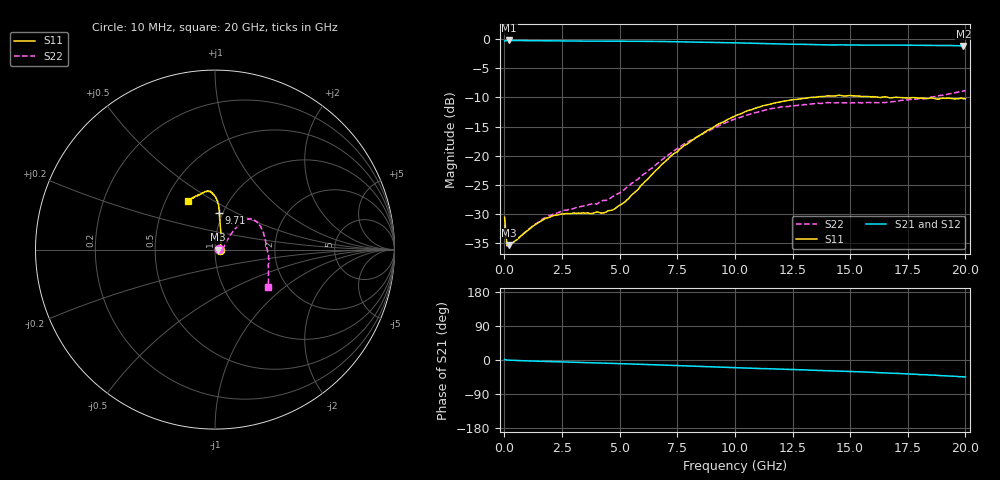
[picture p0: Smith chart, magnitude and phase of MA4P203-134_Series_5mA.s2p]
! AWR Design Environment (9226) Thu Aug 19 14:29:25 2021
! Document = '5mA'
! nPorts: 2, nXvals: 201
# GHz S DB R 50
!Freq DBS11 AngS11 DBS21 AngS21 DBS12 AngS12 DBS22 AngS22
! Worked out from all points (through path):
!   201 points, 10 MHz to 20 GHz, reference 50 ohm
!   highest |S21| = -0.20 dB at 210 MHz (marker M1); lowest = -1.1 dB at 19.91 GHz (marker M2)
!   group delay of S21, straight-line fit = 5.94 ps
!   lowest |S11| = -35.4 dB at 210 MHz (marker M3), VSWR 1.03, Z = 51.7 - j0.00352 ohm
!   |S11| at or under -10 dB: start of sweep to 13.27 GHz; 16.66 GHz to 16.89 GHz (226.5 MHz wide, 1.35 % of centre); 17.13 GHz to end of sweep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
!   |S22| runs from -35.6 to -8.8 dB; largest |S21 - S12| = 0.043
!   S11 on the Smith chart (normalised r, x): 10 MHz: 1.06, -0.00; 9.71 GHz: 0.96, +0.41; 20 GHz: 0.65, +0.39
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0.01  -30.60 -1.1  -0.28 1.4  -0.26 1.0  -31.91 11.3
0.11  -35.35 -2.9  -0.20 -0.2  -0.19 -0.2  -35.56 -3.5
0.21  -35.36 -0.1  -0.20 -0.5  -0.19 -0.5  -35.42 0.5
1.21  -32.21 -4.0  -0.25 -2.7  -0.23 -2.6  -32.14 -4.3
1.81  -30.76 -11.5  -0.28 -3.8  -0.26 -3.5  -30.57 -11.5
2.41  -30.09 -15.8  -0.29 -4.8  -0.28 -4.5  -29.67 -15.9
3.41  -29.83 -10.7  -0.31 -6.7  -0.29 -6.1  -28.66 -11.9
4.01  -29.67 -0.2  -0.31 -7.8  -0.30 -7.2  -28.35 -3.8
4.21  -29.90 6.7  -0.32 -8.1  -0.30 -7.5  -27.79 -1.1
4.81  -29.10 23.8  -0.33 -9.2  -0.31 -8.6  -26.84 8.9
5.31  -27.67 38.7  -0.33 -10.2  -0.32 -9.4  -25.44 18.3
6.71  -22.04 65.5  -0.37 -13.1  -0.34 -12.2  -21.13 38.0
7.81  -18.21 75.6  -0.43 -15.5  -0.42 -14.5  -17.96 44.1
9.71  -13.72 83.3  -0.58 -19.5  -0.57 -18.3  -14.16 46.3
10.01  -13.18 83.5  -0.61 -20.3  -0.60 -18.9  -13.69 46.4
11.21  -11.42 86.6  -0.72 -22.8  -0.72 -21.1  -12.28 43.9
13.41  -9.98 93.5  -0.91 -26.8  -0.87 -25.1  -11.07 34.0
14.51  -9.60 97.1  -0.97 -29.2  -0.91 -27.2  -10.88 26.9
16.71  -10.06 107.7  -0.99 -34.7  -0.92 -32.3  -10.78 2.4
18.21  -10.14 115.9  -1.04 -38.6  -0.94 -37.1  -10.23 -16.3
19.91  -10.21 120.5  -1.12 -44.3  -1.05 -43.1  -8.90 -34.0
20  -10.21 119.3  -1.12 -44.9  -1.05 -43.3  -8.83 -34.9
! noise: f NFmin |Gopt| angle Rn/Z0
0.01  0  1  0  2e-20
2.21  0  1  0  2e-20
4.41  0  1  0  2e-20
6.61  0  1  0  2e-20
8.81  0  1  0  2e-20
11.11  0  1  0  2e-20
13.31  0  1  0  2e-20
15.51  0  1  0  2e-20
17.71  0  1  0  2e-20
20  0  1  0  2e-20
